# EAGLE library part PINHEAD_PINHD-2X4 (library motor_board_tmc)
PIN HEADER
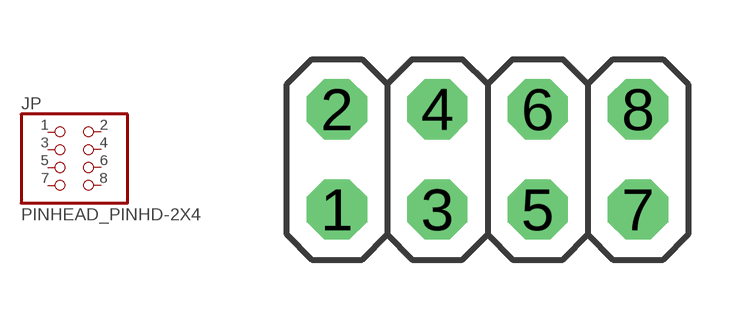
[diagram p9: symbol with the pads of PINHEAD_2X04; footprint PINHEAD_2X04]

Designator prefix JP

## PINHEAD_PINHD-2X4  [PINHEAD_2X04]
1  1  pas
2  2  pas
3  3  pas
4  4  pas
5  5  pas
6  6  pas
7  7  pas
8  8  pas

## Footprint PINHEAD_2X04 (pad centres in mm)
PIN HEADER
drill 1.016 octagon: 1 -3.81,-1.27; 2 -3.81,1.27; 3 -1.27,-1.27; 4 -1.27,1.27; 5 1.27,-1.27; 6 1.27,1.27; 7 3.81,-1.27; 8 3.81,1.27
